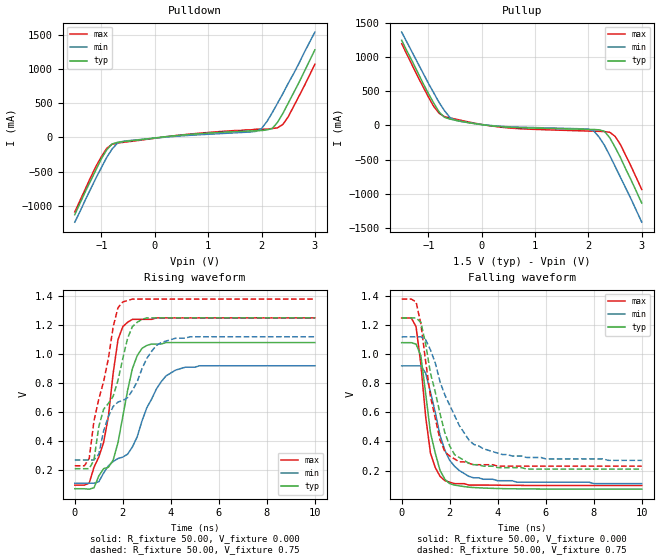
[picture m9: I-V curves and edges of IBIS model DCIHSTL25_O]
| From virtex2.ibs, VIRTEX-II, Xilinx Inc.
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|   Model DCIHSTL25_O
[Model]   DCIHSTL25_O
Model_type   Output
Polarity   Non-Inverting
Vmeas =   0.75V
Cref =  20.00pF
Rref =  50.00
Vref =   0.75V
C_comp   7.00pF   6.00pF   8.00pF
[Temperature Range]   25.00   100.00   0.000
[Voltage Range]   1.50V   1.40V   1.60V
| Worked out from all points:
|   slope of the pulldown table from 0 to 0.225 V, typ, clamps not added: 11 ohm
|   slope of the pullup table from 0 to 0.225 V, typ, clamps not added: 11.1 ohm
|   rising waveform, R_fixture 50.00, V_fixture 0.000: 20-80 % time 765ps typ, 1.67ns min, 655ps max; typ from 0.072 V to 1.08 V
|   rising waveform, R_fixture 50.00, V_fixture 0.75: 20-80 % time 1.17ns typ, 1.78ns min, 825ps max; typ from 0.21 V to 1.25 V
|   falling waveform, R_fixture 50.00, V_fixture 0.000: 20-80 % time 592ps typ, 822ps min, 463ps max; typ from 1.08 V to 0.072 V
|   falling waveform, R_fixture 50.00, V_fixture 0.75: 20-80 % time 865ps typ, 1.3ns min, 687ps max; typ from 1.25 V to 0.21 V
[Pulldown]
| voltage   I(typ)   I(min)   I(max)
-1.5V     -1.13A     -1.24A     -1.09A
-1V       -310mA     -440mA     -280mA
-900mV    -180mA     -290mA     -160mA
-800mV    -95.82mA   -170mA     -100mA
-700mV    -72.67mA   -83.99mA   -83.93mA
300mV     18.39mA    10.36mA    18.29mA
1.8V      94.12mA    79.91mA    110mA
2V        100mA      130mA      120mA
2.2V      130mA      360mA      130mA
2.4V      350mA      640mA      190mA
2.5V      500mA      790mA      300mA
3V        1.28A      1.54A      1.07A
[Pullup]
| voltage   I(typ)   I(min)   I(max)
-1.5V     1.25A      1.37A      1.2A
-900mV    330mA      480mA      280mA
-700mV    120mA      220mA      130mA
-600mV    93.98mA    120mA      110mA
-500mV    77.65mA    77.26mA    95.22mA
500mV     -25.46mA   -19.19mA   -36.42mA
2.1V      -59.79mA   -80.22mA   -84.14mA
2.3V      -86.18mA   -290mA     -90.45mA
2.4V      -180mA     -440mA     -100mA
2.5V      -320mA     -600mA     -160mA
2.6V      -470mA     -760mA     -280mA
3V        -1.14A     -1.42A     -940mA
[Ramp]
| variable   typ   min   max
dV/dt_r   0.60/0.75n   0.48/1.66n   0.69/0.56n
dV/dt_f   0.63/0.97n   0.50/1.68n   0.68/0.75n
R_load = 50.00
[Rising Waveform]
R_fixture = 50.00
V_fixture = 0.000
| time   V(typ)   V(min)   V(max)
0s        71.78mV    110mV      96.67mV
600ps     68.85mV    110mV      110mV
1.2ns     210mV      180mV      390mV
1.6ns     270mV      260mV      870mV
1.8ns     390mV      280mV      1.1V
2.2ns     750mV      310mV      1.22V
2.8ns     1.04V      540mV      1.24V
3.4ns     1.07V      760mV      1.25V
4.2ns     1.08V      890mV      1.25V
10ns      1.08V      920mV      1.25V
[Rising Waveform]
R_fixture = 50.00
V_fixture = 0.75
V_fixture_min = 0.70
V_fixture_max = 0.80
| time   V(typ)   V(min)   V(max)
0s        210mV      270mV      230mV
600ps     210mV      270mV      280mV
800ps     270mV      270mV      540mV
1ns       500mV      310mV      690mV
1.2ns     620mV      470mV      810mV
1.6ns     710mV      640mV      1.19V
2ns       970mV      680mV      1.36V
2.4ns     1.19V      750mV      1.38V
3.6ns     1.25V      1.08V      1.38V
10ns      1.25V      1.12V      1.38V
[Falling Waveform]
R_fixture = 50.00
V_fixture = 0.000
| time   V(typ)   V(min)   V(max)
0s        1.08V      920mV      1.25V
600ps     1.07V      920mV      1.19V
800ps     990mV      920mV      930mV
1ns       730mV      870mV      570mV
1.2ns     460mV      740mV      320mV
1.6ns     200mV      440mV      160mV
1.8ns     140mV      340mV      130mV
2.2ns     100mV      230mV      110mV
3ns       82.91mV    150mV      100mV
10ns      71.84mV    110mV      96.69mV
[Falling Waveform]
R_fixture = 50.00
V_fixture = 0.75
V_fixture_min = 0.70
V_fixture_max = 0.80
| time   V(typ)   V(min)   V(max)
0s        1.25V      1.12V      1.38V
600ps     1.25V      1.12V      1.36V
800ps     1.22V      1.12V      1.21V
1.2ns     870mV      1.03V      710mV
1.6ns     590mV      810mV      410mV
2ns       370mV      650mV      300mV
2.2ns     310mV      580mV      280mV
2.8ns     250mV      410mV      250mV
4.2ns     220mV      310mV      230mV
10ns      210mV      270mV      230mV
